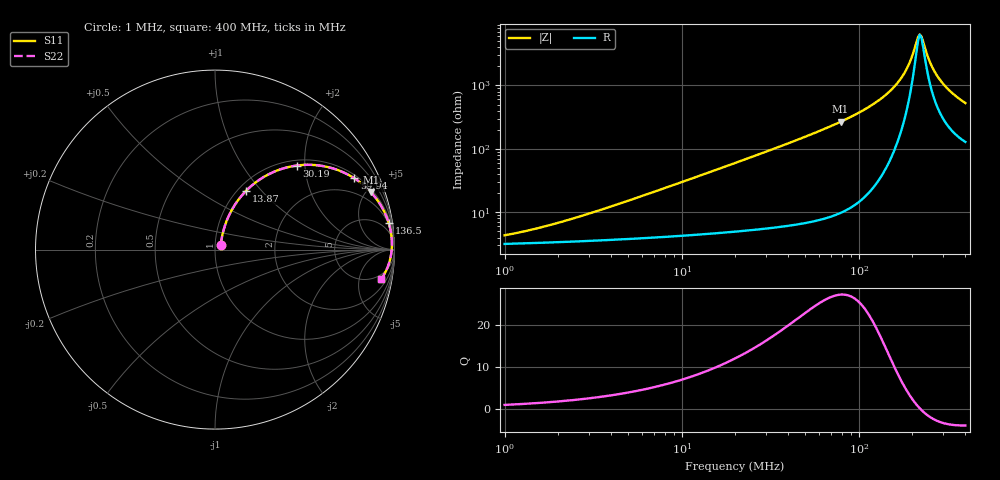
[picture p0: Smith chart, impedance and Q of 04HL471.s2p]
! Coilcraft 0402HL-471 Chip Inductor
! 20 July 2012
# MHz S MA R 50
!Freq  MagS11  AngS11  MagS21  AngS21  MagS12  AngS12  MagS22  AngS22
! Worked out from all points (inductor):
!   263 points, 1 MHz to 400 MHz, reference 50 ohm
!   read as one part in series: L = 470 nH near 3.767 MHz
!   highest Q = 27.3 at 78.87 MHz (marker M1), where L = 538 nH
!   self-resonance near 220.7 MHz
!   S11 on the Smith chart (normalised r, x): 1 MHz: 1.06, +0.06; 13.87 MHz: 1.09, +0.82; 30.19 MHz: 1.11, +1.82; 59.94 MHz: 1.15, +3.82; 136.5 MHz: 2, +13; 400 MHz: 4, -10
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1  0.04198 41.3  0.9689 -1.6  0.9689 -1.6  0.04198 41.3
2.735188  0.0848 62.1  0.9633 -4.5  0.9633 -4.5  0.0848 62.1
7.481253  0.2114 67.6  0.9402 -12.0  0.9402 -12.0  0.2114 67.6
13.87157  0.3683 62.2  0.8901 -21.5  0.8901 -21.5  0.3683 62.2
20  0.4952 55.7  0.8287 -29.6  0.8287 -29.6  0.4952 55.7
30.18544  0.6535 45.8  0.7182 -40.7  0.7182 -40.7  0.6535 45.8
54.70376  0.8496 29.5  0.4935 -58.1  0.4935 -58.1  0.8496 29.5
59.94366  0.872 27.1  0.4562 -60.6  0.4562 -60.6  0.872 27.1
78.87177  0.9254 20.3  0.3468 -67.6  0.3468 -67.6  0.9254 20.3
106.1772  0.962 13.7  0.2364 -74.0  0.2364 -74.0  0.962 13.7
136.5458  0.9792 8.7  0.1509 -77.8  0.1509 -77.8  0.9792 8.7
149.6251  0.9829 7.0  0.1215 -78.4  0.1215 -78.4  0.9829 7.0
167.7498  0.9857 4.9  0.08583 -77.9  0.08583 -77.9  0.9857 4.9
183.818  0.9865 3.3  0.05828 -75.0  0.05828 -75.0  0.9865 3.3
196.8714  0.9864 2.1  0.03853 -68.3  0.03853 -68.3  0.9864 2.1
215.7291  0.9851 0.5  0.01728 -30.5  0.01728 -30.5  0.9851 0.5
220.7193  0.9846 0.1  0.01549 -7.6  0.01549 -7.6  0.9846 0.1
225.8249  0.9841 -0.3  0.0166 16.2  0.0166 16.2  0.9841 -0.3
253.18  0.98 -2.2  0.04305 61.3  0.04305 61.3  0.98 -2.2
277.4314  0.9753 -3.8  0.06923 67.2  0.06923 67.2  0.9753 -3.8
325.5939  0.9636 -6.5  0.1165 68.6  0.1165 68.6  0.9636 -6.5
400  0.9414 -10.0  0.1786 65.9  0.1786 65.9  0.9414 -10.0
